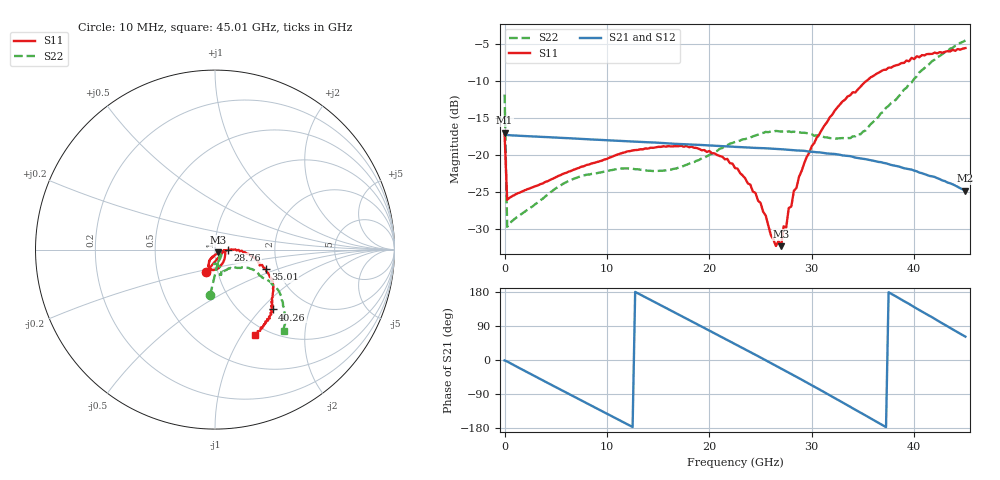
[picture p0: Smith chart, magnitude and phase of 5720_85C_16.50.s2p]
! Device:  ADRF5720
! Description: 0.5dB LSB GaAs MMIC 6-bit Digital Attenuator
! Frequency:  0.000009 -  40 GHz
! Ports:
!	RF1	= Port 1
!	RF2	= Port 2
! Vdd:  3.3 Volt
! Vss:  -3.3 Volt
! Control:  0/3.3 Volt
! State:  16.50 dB attenuation
! Data:  The device was measured using G-S-G Probes on a matrix board.
!  Data was collected using an calibrated 4 port network analyzer.
!  The reference plane for this measurement is at the launchers.
! Note:  Analog Devices supplies this data as a sample of measured data
!  for this product.  Your particular data for this product may vary.
!  Data was taken at 85 degrees C.
!  Analog Devices reserves the right to change this data at anytime.
# GHZ S DB R 45.0
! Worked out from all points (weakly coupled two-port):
!   181 points, 10 MHz to 45.01 GHz, reference 45 ohm
!   highest |S21| = -17.01 dB at 10 MHz (marker M1); lowest = -24.8 dB at 45.01 GHz (marker M2)
!   lowest |S11| = -32.3 dB at 27.01 GHz (marker M3), VSWR 1.05, Z = 46.7 - j1.4 ohm
!   |S11| at or under -10 dB: start of sweep to 35.36 GHz
!   |S22| runs from -29.7 to -4.6 dB; largest |S21 - S12| = 0.00066
!   S11 on the Smith chart (normalised r, x): 10 MHz: 0.88, -0.23; 28.76 GHz: 1.15, -0.00; 35.01 GHz: 1.73, -0.40; 40.26 GHz: 1.37, -1.17; 45.01 GHz: 0.87, -1.14
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0.01  -17.26 -111.9  -17.01 -1.2  -17.00 -1.2  -11.86 -96.2
0.26  -26.07 -10.4  -17.32 -3.9  -17.32 -3.9  -29.71 -15.4
4.26  -23.53 -33.9  -17.61 -61.1  -17.60 -61.1  -25.32 -55.5
7.76  -21.53 -57.1  -17.86 -110.3  -17.85 -110.2  -22.77 -80.0
11.51  -19.74 -77.3  -18.13 -162.8  -18.12 -162.7  -21.83 -92.8
15.26  -18.92 -93.0  -18.38 144.4  -18.37 144.6  -22.14 -89.5
20.01  -19.48 -108.6  -18.72 77.5  -18.71 77.7  -20.01 -74.3
22.76  -21.86 -113.8  -18.93 38.6  -18.92 38.8  -18.16 -73.3
25.01  -26.49 -107.8  -19.08 6.5  -19.07 6.8  -17.13 -76.2
26.51  -32.29 -65.5  -19.19 -15.2  -19.18 -15.0  -16.77 -76.5
27.01  -32.32 -38.3  -19.23 -22.5  -19.21 -22.3  -16.85 -76.7
27.26  -29.64 -26.1  -19.26 -26.3  -19.25 -26.0  -16.83 -77.4
27.51  -29.78 -17.1  -19.29 -29.9  -19.28 -29.6  -16.92 -77.0
27.76  -27.18 -11.8  -19.31 -33.5  -19.30 -33.2  -16.82 -77.8
28.01  -26.95 -8.4  -19.35 -37.2  -19.33 -36.9  -16.92 -77.5
28.76  -22.97 -1.5  -19.42 -48.0  -19.41 -47.7  -16.95 -77.9
30.26  -18.38 -2.2  -19.61 -70.3  -19.59 -70.0  -17.42 -76.0
32.26  -14.01 -9.3  -19.88 -100.4  -19.87 -100.1  -17.82 -66.9
35.01  -10.42 -20.7  -20.51 -142.5  -20.50 -142.2  -16.86 -45.3
37.76  -8.23 -33.6  -21.36 174.9  -21.34 175.3  -13.01 -28.6
40.26  -6.69 -46.1  -22.22 135.6  -22.20 136.1  -9.40 -30.1
45.01  -5.59 -65.0  -24.83 61.7  -24.81 61.9  -4.56 -49.8
